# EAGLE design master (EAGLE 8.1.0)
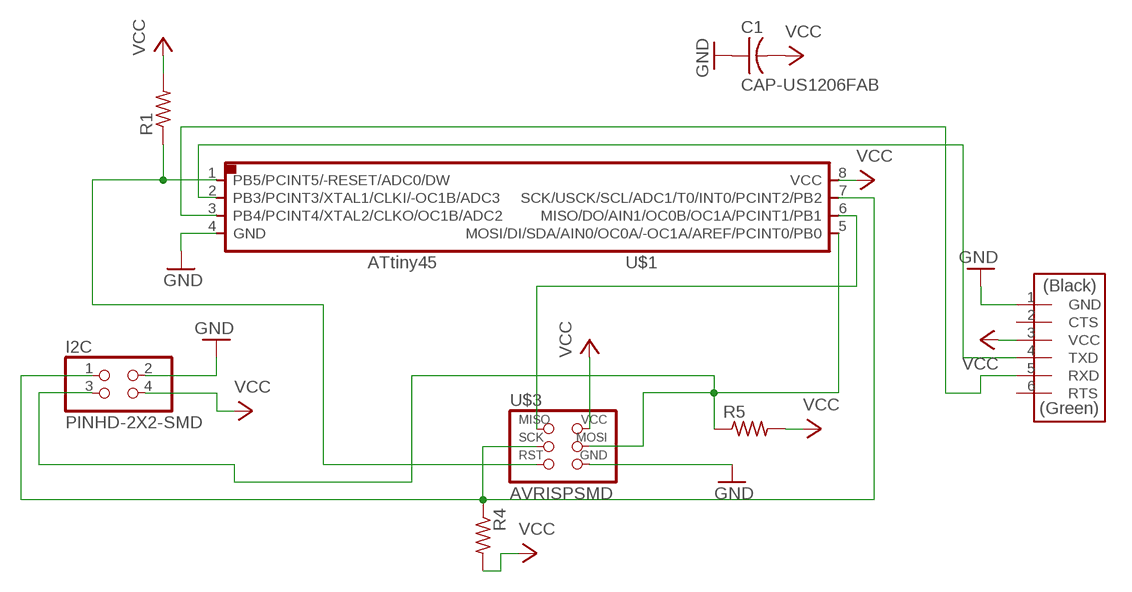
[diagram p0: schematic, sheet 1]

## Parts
C1  CAP-US1206FAB  [C1206FAB]
I2C  PINHD-2X2-SMD  [2X02SMD]
R1  RES-US1206FAB  [R1206FAB]
R4  RES-US1206FAB  [R1206FAB]
R5  RES-US1206FAB  [R1206FAB]
U$1  ATTINY45SI  [SOIC8]
U$2  FTDI-SMD-HEADER  [1X06SMD]
U$3  AVRISPSMD  [2X03SMD]

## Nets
GND: C1.1 I2C.2 U$1.4(GND) U$2.1(GND) U$3.6(GND)
N$1: R1.1 U$1.1(PB5/PCINT5/-RESET/ADC0/DW) U$3.5(RST)
N$2: U$1.6(MISO/DO/AIN1/OC0B/OC1A/PCINT1/PB1) U$3.1(MISO)
N$3: I2C.3 R5.1 U$1.5(MOSI/DI/SDA/AIN0/OC0A/-OC1A/AREF/PCINT0/PB0) U$3.4(MOSI)
N$4: I2C.1 R4.1 U$1.7(SCK/USCK/SCL/ADC1/T0/INT0/PCINT2/PB2) U$3.3(SCK)
N$5: U$1.2(PB3/PCINT3/XTAL1/CLKI/-OC1B/ADC3) U$2.4(TXD)
N$6: U$1.3(PB4/PCINT4/XTAL2/CLKO/OC1B/ADC2) U$2.5(RXD)
VCC: C1.2 I2C.4 R1.2 R4.2 R5.2 U$1.8(VCC) U$2.3(VCC) U$3.2(VCC)
Unconnected: U$2.2(CTS) U$2.6(RTS)

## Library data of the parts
C1 = fab:CAP-US
I2C = fab:PINHD-2X2-SMD
R1 R4 R5 = fab:RES-US: Resistor (US Symbol)
U$1 = fab:ATTINY45
U$2 = fab:FTDI-SMD-HEADER
U$3 = fab:AVRISP

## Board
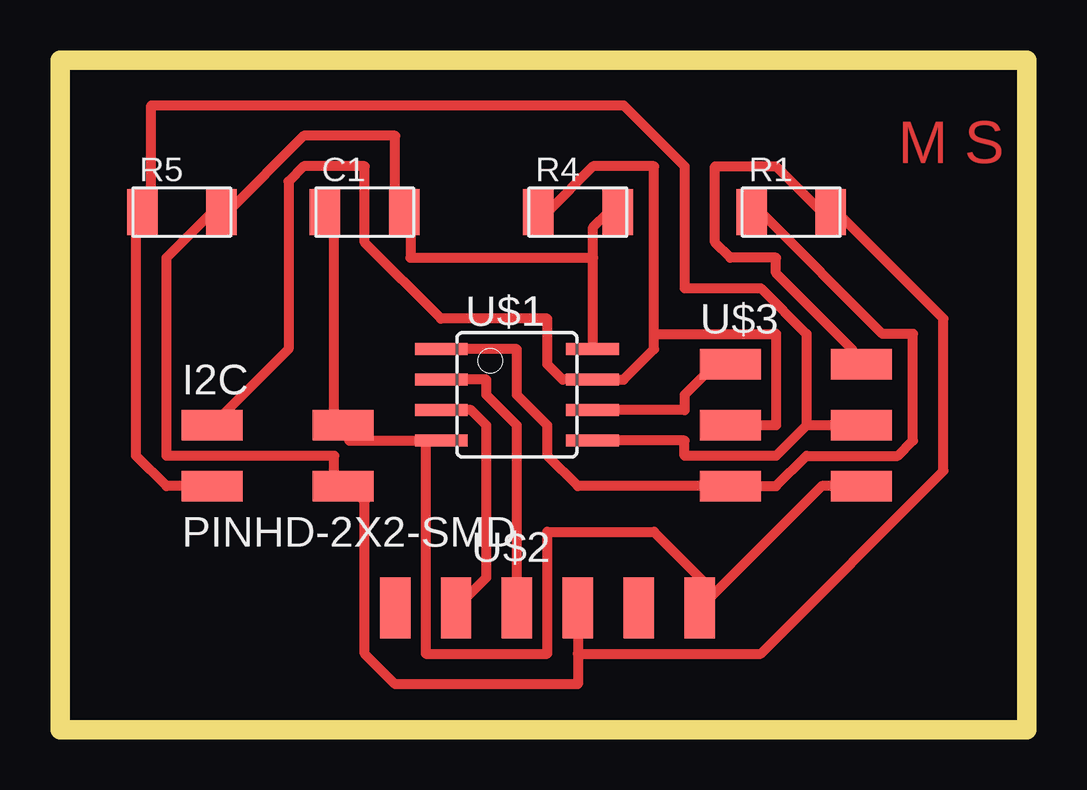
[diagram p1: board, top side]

Size 40.31 x 27.93 mm. Coordinates in mm from the lower left corner, seen from the top.
Outline: 0,0 40.31,0 40.31,27.93 0,27.93 0,0
Copper layers (1*16): Top 0.035mm / dielectric 1.5mm / Bottom 0.035mm
Design rules "default *": minimum track width 16mil, minimum drill 24mil, track to track 16mil, track to pad 16mil, pad to pad 16mil, via to via 16mil, smd to smd 8mil, copper to edge 40mil, drill to drill 8mil, minimum pad ring 10mil, minimum via ring 8mil, stop-mask expansion 4mil, vias tented up to drill 0mil, thermal gap 10mil

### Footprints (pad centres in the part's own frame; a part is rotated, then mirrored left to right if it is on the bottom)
C1206FAB = smd 1.27 x 1.905: 1 -1.651,0; 2 1.651,0
2X02SMD = smd 2.54 x 1.27: 1 -2.54,1.27; 2 2.92,1.27; 3 -2.54,-1.27; 4 2.92,-1.27
R1206FAB = smd 1.27 x 1.905: 1 -1.651,0; 2 1.651,0
SOIC8 = smd 0.5 x 2.2: 1 -1.905,-3.154; 2 -0.645,-3.154; 3 0.625,-3.154; 4 1.895,-3.154; 5 1.905,3.154; 6 0.635,3.154; 7 -0.635,3.154; 8 -1.905,3.154
1X06SMD = smd 2.54 x 1.27: 1 0,6.35; 2 0,3.81; 3 0,1.27; 4 0,-1.27; 5 0,-3.81; 6 0,-6.35
2X03SMD = smd 2.54 x 1.27: 1 -2.54,2.54; 2 2.92,2.54; 3 -2.54,0; 4 2.92,0; 5 -2.54,-2.54; 6 2.92,-2.54

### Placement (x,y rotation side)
C1  12.7,21.59 0 top
I2C  8.89,11.43 0 top
R1  30.48,21.59 0 top
R4  21.59,21.59 0 top
R5  5.08,21.59 0 top
U$1  19.05,13.97 270 top
U$2  20.32,5.08 270 top
U$3  30.48,12.7 0 top

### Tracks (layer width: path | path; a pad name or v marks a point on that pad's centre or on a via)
GND
  Top 0.406: 27.3,5.72 31.75,10.16 U$3.6 | 27.3,5.72 U$2.1 | C1.1 11.43,21.59 11.43,12.7 I2C.2 12.06,12.7 12.06,12.07 15.24,12.07 | 15.24,12.07 15.88,12.07 U$1.4 15.24,12.07 | 27.3,5.72 24.77,8.26 20.32,8.26 20.32,3.18 15.24,3.18 15.24,12.07
N$1
  Top 0.406: R1.1 29.21,21.59 34.29,16.51 35.56,16.51 35.56,12.07 34.92,11.43 31.11,11.43 29.84,10.16 U$3.5 21.59,10.16 20.32,11.43 20.32,12.7 19.05,13.97 19.05,15.88 U$1.1
N$2
  Top 0.406: U$1.6 26.03,13.34 26.03,13.97 27.3,15.24 U$3.1
N$3
  Top 0.406: U$1.5 26.03,12.07 26.03,11.43 29.84,11.43 31.11,12.7 | U$3.4 31.11,12.7 | I2C.3 4.44,10.16 3.17,11.43 3.17,21.59 R5.1 3.81,21.59 3.81,26.04 23.49,26.04 26.03,23.5 26.03,18.41 29.21,18.41 31.11,16.51 31.11,12.7
N$4
  Top 0.406: 24.77,16.51 24.77,15.88 23.49,14.61 U$1.7 20.95,14.61 20.32,15.24 20.32,17.15 15.88,17.15 12.7,20.32 12.7,23.5 10.16,23.5 9.52,22.86 9.52,15.88 I2C.1 | 24.77,16.51 24.77,23.5 22.23,23.5 20.32,21.59 R4.1 | U$3.3 29.84,12.7 29.84,16.51 24.77,16.51
N$5
  Top 0.406: U$2.4 19.05,12.7 17.78,13.97 17.78,14.61 16.51,14.61 U$1.2
N$6
  Top 0.406: U$2.5 17.78,6.35 17.78,12.7 17.14,13.34 16.51,13.34 U$1.3
VCC
  Top 0.406: 22.23,19.69 22.23,15.88 U$1.8 | 22.23,19.69 22.23,20.95 22.86,21.59 R4.2 | 22.23,19.69 14.6,19.69 14.6,21.59 C1.2 13.97,21.59 13.97,24.77 10.16,24.77 6.98,21.59 R5.2 6.35,21.59 4.44,19.69 4.44,11.43 11.43,11.43 11.43,10.16 I2C.4 12.06,10.16 12.7,9.52 12.7,3.18 13.97,1.91 21.59,1.91 21.59,3.18 | U$3.2 33.02,15.24 33.02,15.88 29.84,19.05 29.84,19.69 27.94,19.69 27.3,20.32 27.3,23.5 29.84,23.5 31.75,21.59 R1.2 32.38,21.59 36.83,17.15 36.83,10.8 29.21,3.18 21.59,3.18 | U$2.3 21.59,3.18

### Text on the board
Top: M S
